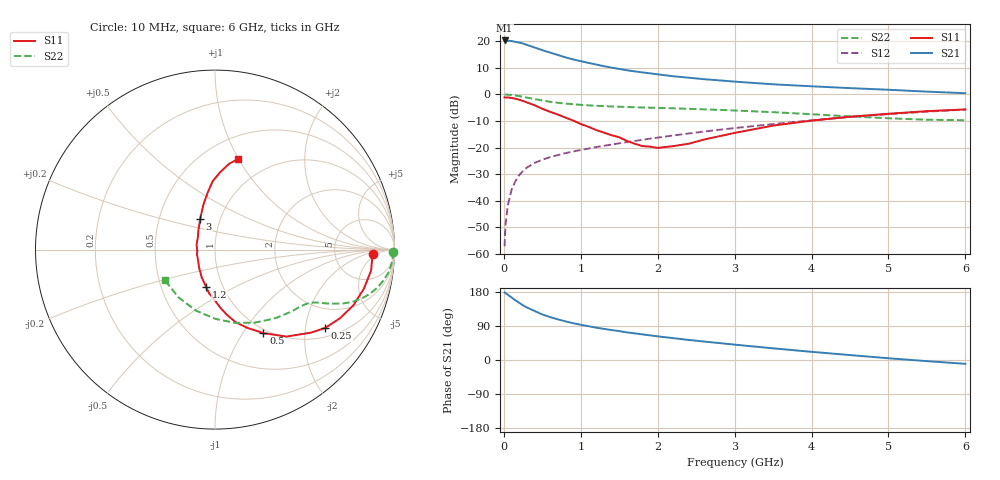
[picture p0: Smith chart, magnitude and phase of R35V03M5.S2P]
! SIEMENS Small Signal Semiconductors
! BFR181
! Si NPN RF Bipolar Junction Transistor in SOT23
! VCE = 5 V  IC = 3.5 mA
! Common Emitter S-Parameters:  May  1996
# GHz  S  MA  R  50
!  f  S11  S21  S12  S22
! GHz  MAG  ANG  MAG  ANG  MAG  ANG  MAG  ANG
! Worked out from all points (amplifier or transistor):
!   36 points, 10 MHz to 6 GHz, reference 50 ohm
!   highest |S21| = 20.3 dB at 10 MHz (marker M1)
!   |S21| within 3 dB of that: start of sweep to 434.8 MHz
!   unconditionally stable (mu >= 1): 1.324 GHz to 3.168 GHz
!   at 250 MHz: K = 0.33, MSG = 24.0 dB, |S12| = -28.8 dB
!   at 1.4 GHz: K = 1.02, MAG = 13.7 dB, |S12| = -18.9 dB
!   at 6 GHz: K = 0.86, MSG = 3.1 dB, |S12| = -5.7 dB
!   S11 on the Smith chart (normalised r, x): 10 MHz: 15, -4; 250 MHz: 1.27, -2.56; 500 MHz: 0.95, -1.24; 1.2 GHz: 0.83, -0.36; 3 GHz: 0.80, +0.28; 6 GHz: 0.72, +1.00
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0.01  0.8828 -1.7  10.37 178.3  0.0014 92.7  0.9939 -0.7
0.02  0.8772 -2.9  10.18 176.6  0.0033 85.8  0.9924 -1.5
0.05  0.8776 -7.6  10.2 172.4  0.008 85.9  0.9898 -3.6
0.1  0.8578 -14.7  10.14 165.3  0.016 82.1  0.9783 -7.1
0.15  0.8313 -21.9  9.731 157.4  0.0234 77.6  0.9553 -10.2
0.2  0.7944 -28.8  9.459 150.8  0.0305 74.4  0.9317 -13.0
0.25  0.7527 -35.5  9.085 144.2  0.0364 70.9  0.9014 -15.6
0.3  0.7067 -40.9  8.539 138.6  0.0421 69.1  0.8723 -17.7
0.4  0.6269 -50.6  7.641 129.4  0.0516 65.4  0.8196 -20.8
0.5  0.538 -59.9  6.804 120.1  0.0592 62.7  0.7701 -23.0
0.6  0.4716 -67.6  6.14 113.3  0.0663 61.5  0.7284 -24.4
0.8  0.3674 -79.9  4.989 102.0  0.0786 59.9  0.6739 -26.3
0.9  0.3239 -84.9  4.565 97.1  0.0846 59.8  0.6546 -26.9
1.1  0.2467 -97.5  3.926 89.2  0.096 60.2  0.6231 -28.3
1.2  0.2145 -103.3  3.655 85.3  0.1024 60.5  0.6119 -28.9
1.6  0.1335 -131.7  2.853 72.9  0.1268 60.7  0.581 -32.2
2.2  0.1065 164.9  2.2 57.7  0.1689 60.4  0.5487 -38.9
3  0.1888 116.1  1.743 40.5  0.233 57.2  0.4996 -50.8
3.5  0.2593 104.4  1.553 30.8  0.2774 53.7  0.4641 -61.2
4.5  0.3815 91.9  1.315 13.0  0.3761 44.3  0.386 -89.7
5.5  0.4849 80.6  1.13 -3.0  0.4746 31.9  0.3347 -127.6
6  0.5227 75.5  1.056 -10.1  0.5194 24.9  0.3274 -148.6
